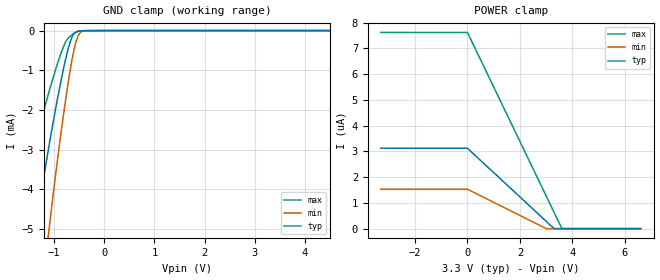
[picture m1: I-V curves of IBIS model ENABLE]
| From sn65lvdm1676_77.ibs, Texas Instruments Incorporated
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|   Input  Model
[Model]   ENABLE
Model_type   Input
|Signals   ATX/RX,BTX/RX,CTX/RX,DTX/RX
Vinh = 2.0
Vinl = 0.8
|   typ   min   max
C_comp   1.279pF   1.192pF   1.306pF
|   typ   min   max
| Junction Temperature (Ambient temp is 25C typ, 85C min, 0C max)
[Temperature Range]   40   100   -40
[Voltage range]   3.3V   3.0   3.6
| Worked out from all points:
|   GND clamp passes 1 mA (typ) near -0.82 V on its own axis
[GND Clamp]
|   Voltage   I(typ)   I(min)   I(max)
-3.3V     -25.81mA   -38.44mA   -16.11mA
-1.762V   -8.443mA   -13.14mA   -5.021mA
-1.389V   -5.166mA   -8.34mA    -2.938mA
-1.365V   -4.962mA   -8.04mA    -2.81mA
-1.117V   -3.022mA   -5.192mA   -1.615mA
-1.092V   -2.839mA   -4.923mA   -1.505mA
-918mV    -1.627mA   -3.128mA   -780uA
-744.4mV  -586uA     -1.527mA   -233.6uA
-645.1mV  -173.2uA   -755.1uA   -108.7uA
-545.9mV  -26.71uA   -212.3uA   -32.46uA
-347.4mV  -1.277uA   -1.846uA   -2.479uA
6.6V      0A         0A         0A
[POWER Clamp]
|   Voltage   I(typ)   I(min)   I(max)
-3.3V     3.126uA    1.534uA    7.625uA
0V        3.124uA    1.533uA    7.622uA
3.002V    281.9nA    0A         1.262uA
3.3V      0A         0A         630.8nA
3.598V    0A         0A         0A
6.6V      0A         0A         0A
